FUNCTION "FC_GRP_81_R29" : VOID
TITLE =GROUP =81-R29
{ S7_language := '9(1) Angielski (Stany Zjednoczone)  11.01.2022  09:45:15' }
VERSION : 0.1


VAR_TEMP
  CL : "UDT_CABINET";	//CABINET LOCAL
  CR : "UDT_CABINET";	//CABINET REMOTE
  RelError : BOOL ;	//ERROR RELEASE
  RelErrorCL : BOOL ;	//ERROR RELEASE FROM CABINET LOCAL
  RelErrorCR : BOOL ;	//ERROR RELEASE FROM CABINET REMOTE
  RelControl : BOOL ;	//CONTROL RELEASE
  RelControlCL : BOOL ;	//CONTROL RELEASE FROM CABINET LOCAL
  RelControlCR : BOOL ;	//CONTROL RELEASE FROM CABINET REMOTE
  ErrorConfirm : BOOL ;	//ERROR CONFIRM
  AutoOn : BOOL ;	//AUTOMATIC ON
  AutoOff : BOOL ;	//AUTOMATIC OFF
  LAMP_ON : BOOL ;
  Setpoint_81FAN72_reached : BOOL ;
  Setpoint_81FAN72_div : BOOL ;
END_VAR
BEGIN
NETWORK
TITLE =GLOBAL SIGNALS
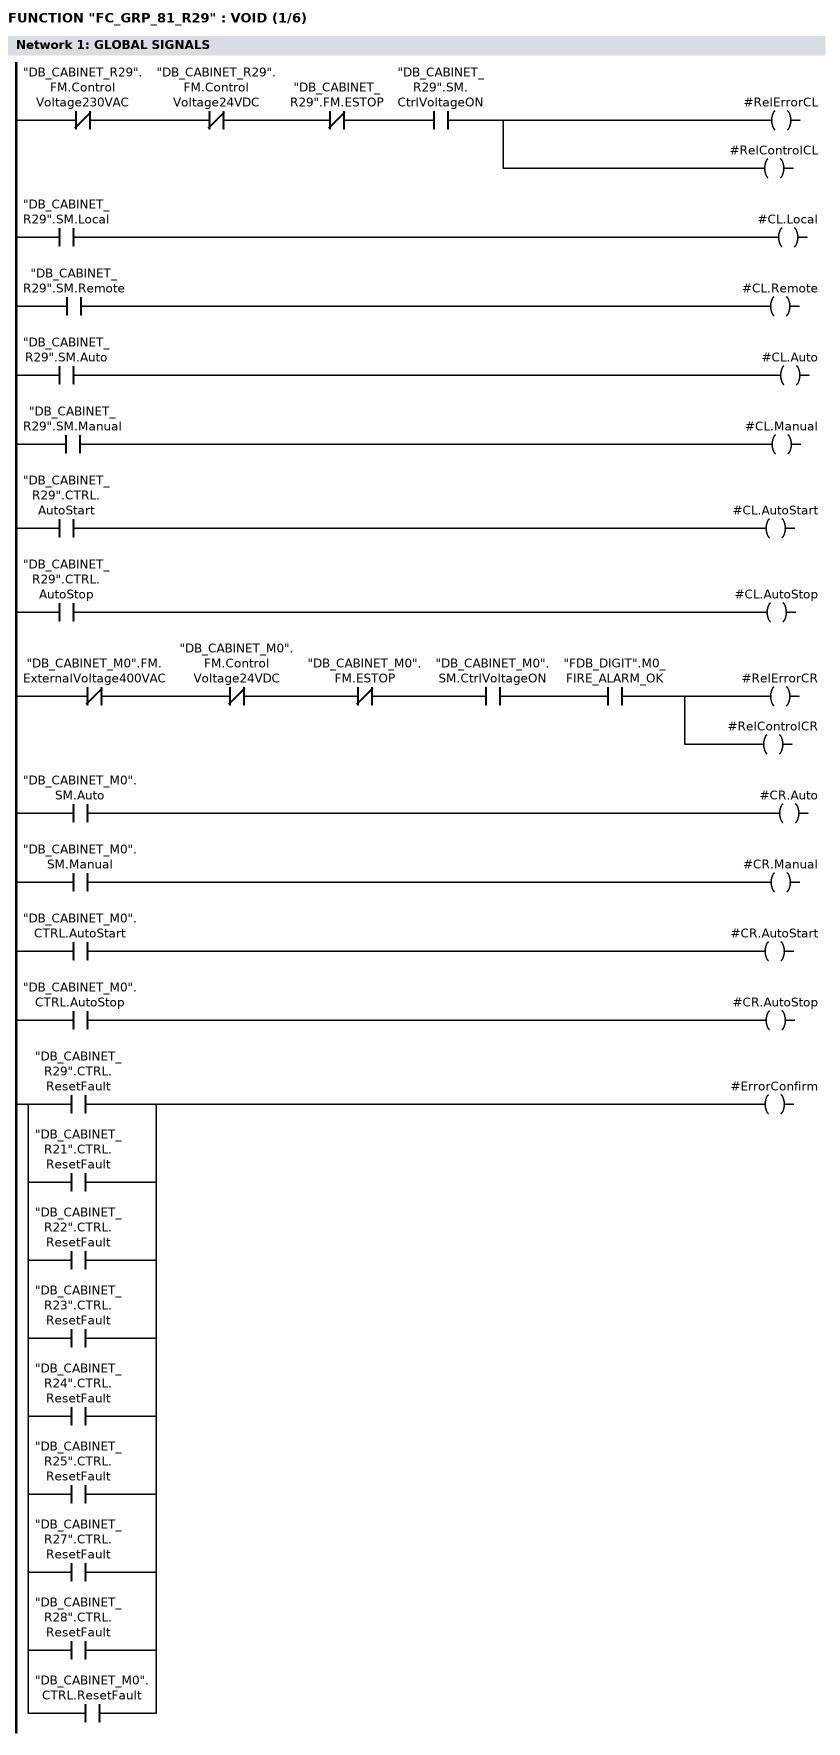
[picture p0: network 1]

// LOCAL
      UN    "DB_CABINET_R29".FM.ControlVoltage230VAC;
      UN    "DB_CABINET_R29".FM.ControlVoltage24VDC;
//      UN    "DB_CABINET_R29".FM.ControlVoltage230VAC_MS
      UN    "DB_CABINET_R29".FM.ESTOP;
      U     "DB_CABINET_R29".SM.CtrlVoltageON;
      =     #RelErrorCL;
      =     #RelControlCL;


      U     "DB_CABINET_R29".SM.Local;
      =     #CL.Local;
      U     "DB_CABINET_R29".SM.Remote;
      =     #CL.Remote;
      U     "DB_CABINET_R29".SM.Auto;
      =     #CL.Auto;
      U     "DB_CABINET_R29".SM.Manual;
      =     #CL.Manual;
      U     "DB_CABINET_R29".CTRL.AutoStart;
      =     #CL.AutoStart;
      U     "DB_CABINET_R29".CTRL.AutoStop;
      =     #CL.AutoStop;

// REMOTE
      UN    "DB_CABINET_M0".FM.ExternalVoltage400VAC;
      UN    "DB_CABINET_M0".FM.ControlVoltage24VDC;
//      UN    "DB_CABINET_M0".FM.ControlVoltage230VAC_MS
      UN    "DB_CABINET_M0".FM.ESTOP;
      U     "DB_CABINET_M0".SM.CtrlVoltageON;
      U     "FDB_DIGIT".M0_FIRE_ALARM_OK;
      =     #RelErrorCR;
      =     #RelControlCR;

      U     "DB_CABINET_M0".SM.Auto;
      =     #CR.Auto;
      U     "DB_CABINET_M0".SM.Manual;
      =     #CR.Manual;
      U     "DB_CABINET_M0".CTRL.AutoStart;
      =     #CR.AutoStart;
      U     "DB_CABINET_M0".CTRL.AutoStop;
      =     #CR.AutoStop;

      U     "DB_CABINET_R29".CTRL.ResetFault;
      O     "DB_CABINET_R21".CTRL.ResetFault;
      O     "DB_CABINET_R22".CTRL.ResetFault;
      O     "DB_CABINET_R23".CTRL.ResetFault;
      O     "DB_CABINET_R24".CTRL.ResetFault;
      O     "DB_CABINET_R25".CTRL.ResetFault;
      O     "DB_CABINET_R27".CTRL.ResetFault;
      O     "DB_CABINET_R28".CTRL.ResetFault;
      O     "DB_CABINET_M0".CTRL.ResetFault;
      =     #ErrorConfirm;

NETWORK
TITLE ==81FAN72-U1 CONTROL/ERROR RELEASE
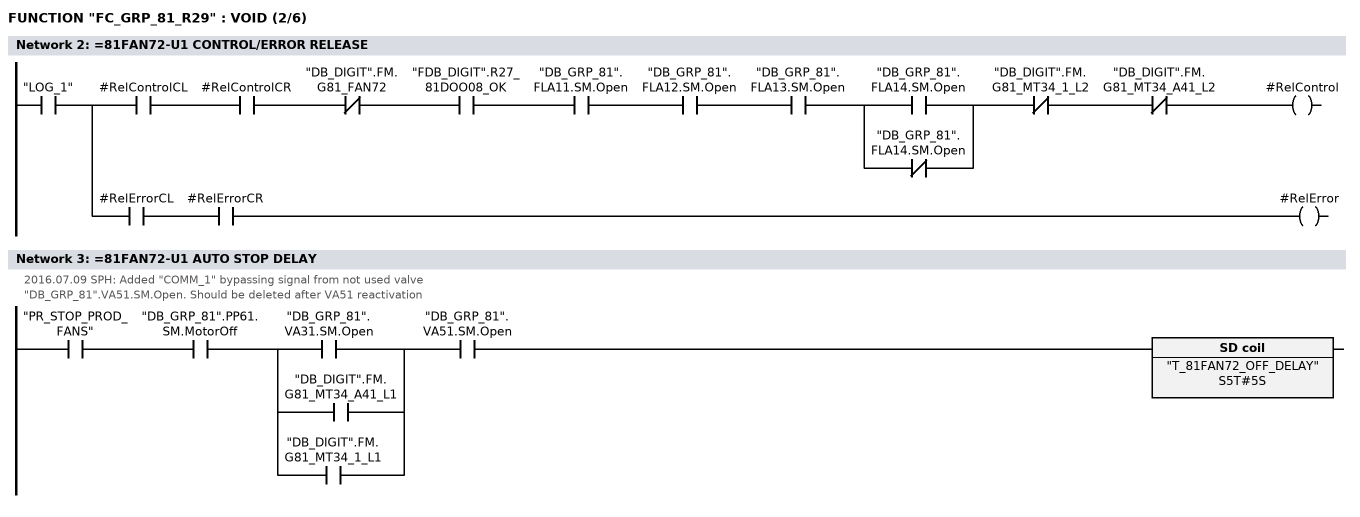
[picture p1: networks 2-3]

      U     "LOG_1";
      =     L      6.0;
      U     L      6.0;
      U     #RelControlCL;
      U     #RelControlCR;
      UN    "DB_DIGIT".FM.G81_FAN72;
      U     "FDB_DIGIT".R27_81DOO08_OK;
      U     "DB_GRP_81".FLA11.SM.Open;
      U     "DB_GRP_81".FLA12.SM.Open;
      U     "DB_GRP_81".FLA13.SM.Open;
      U(    ;
      O     "DB_GRP_81".FLA14.SM.Open;
      ON    "DB_GRP_81".FLA14.SM.Open;
      )     ;
      UN    "DB_DIGIT".FM.G81_MT34_1_L2;
      UN    "DB_DIGIT".FM.G81_MT34_A41_L2;
      =     #RelControl;
      U     L      6.0;
      U     #RelErrorCL;
      U     #RelErrorCR;
      =     #RelError;
NETWORK
TITLE ==81FAN72-U1 AUTO STOP DELAY
//2016.07.09 SPH: Added "COMM_1" bypassing signal from not used valve
//"DB_GRP_81".VA51.SM.Open. Should be deleted after VA51 reactivation
      U     "PR_STOP_PROD_FANS";
      U     "DB_GRP_81".PP61.SM.MotorOff;
      U(    ;
      O     "DB_GRP_81".VA31.SM.Open;
      O     "DB_DIGIT".FM.G81_MT34_A41_L1;
      O     "DB_DIGIT".FM.G81_MT34_1_L1;
      )     ;
      U     "DB_GRP_81".VA51.SM.Open;
      L     S5T#5S;
      SE    "T_81FAN72_OFF_DELAY";
      NOP   0;
      NOP   0;
      NOP   0;
      NOP   0;
NETWORK
TITLE ==81FAN72-U1 CONTROL SIGNALS
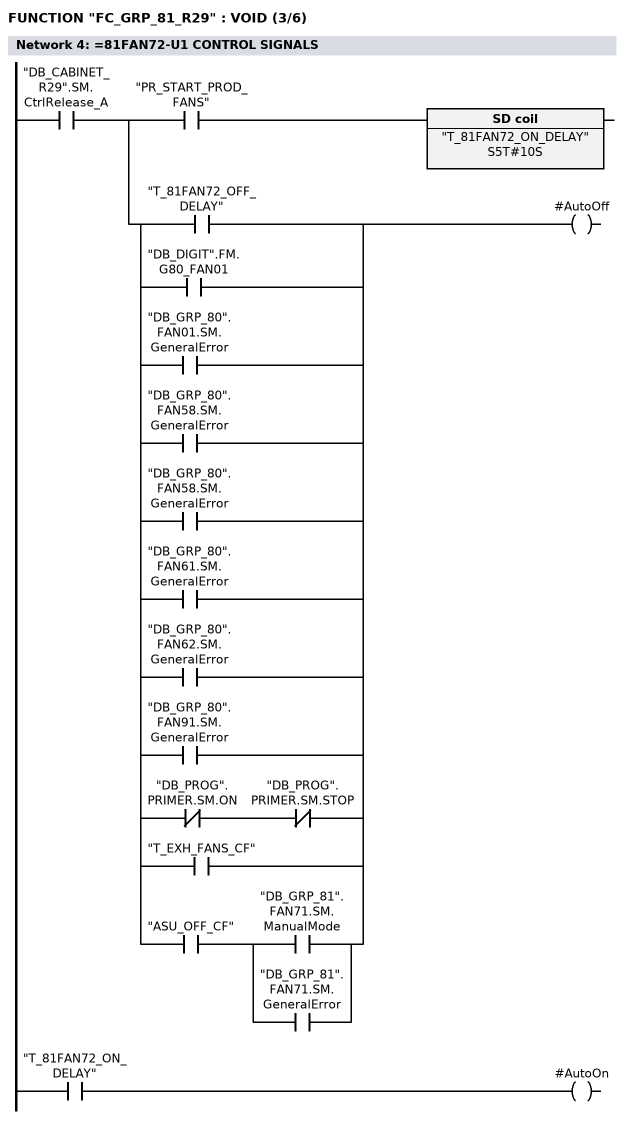
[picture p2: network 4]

      U     "DB_CABINET_R29".SM.CtrlRelease_A;
      =     L      6.0;
      U     L      6.0;
      U     "PR_START_PROD_FANS";
      L     S5T#10S;
      SE    "T_81FAN72_ON_DELAY";
      NOP   0;
      NOP   0;
      NOP   0;
      U     "T_81FAN72_ON_DELAY";
      =     #AutoOn;
      U     L      6.0;
      U(    ;
      O     "T_81FAN72_OFF_DELAY";
      O     "DB_DIGIT".FM.G80_FAN01;
      O     "DB_GRP_80".FAN01.SM.GeneralError;
      O     "DB_GRP_80".FAN58.SM.GeneralError;
      O     "DB_GRP_80".FAN58.SM.GeneralError;
      O     "DB_GRP_80".FAN61.SM.GeneralError;
      O     "DB_GRP_80".FAN62.SM.GeneralError;
      O     "DB_GRP_80".FAN91.SM.GeneralError;
      O     ;
      UN    "DB_PROG".PRIMER.SM.ON;
      UN    "DB_PROG".PRIMER.SM.STOP;
      O     "T_EXH_FANS_CF";
      O     ;
      U     "ASU_OFF_CF";
      U(    ;
      O     "DB_GRP_81".FAN71.SM.ManualMode;
      O     "DB_GRP_81".FAN71.SM.GeneralError;
      )     ;
      )     ;
      =     #AutoOff;
NETWORK
TITLE =SET POINT
//2.800000e+001
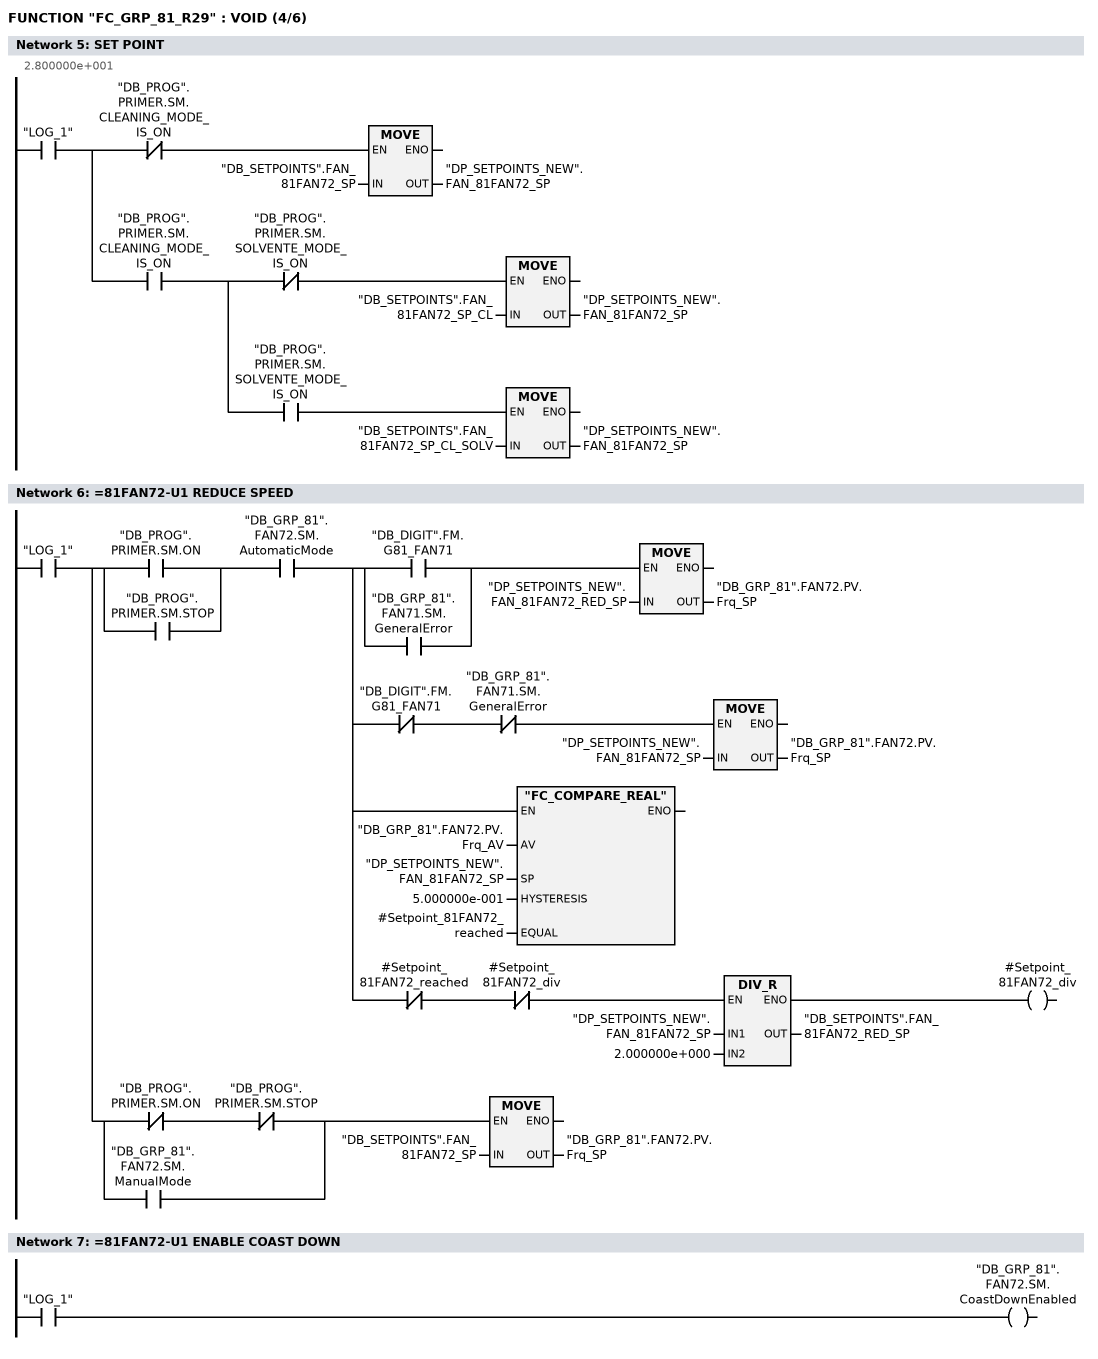
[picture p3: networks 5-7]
      U     "LOG_1";
      =     L      6.0;
      U     L      6.0;
      UN    "DB_PROG".PRIMER.SM.CLEANING_MODE_IS_ON;
      SPBNB _001;
      L     "DB_SETPOINTS".FAN_81FAN72_SP;
      T     "DP_SETPOINTS_NEW".FAN_81FAN72_SP;
_001: NOP   0;
      U     L      6.0;
      U     "DB_PROG".PRIMER.SM.CLEANING_MODE_IS_ON;
      =     L      6.1;
      U     L      6.1;
      UN    "DB_PROG".PRIMER.SM.SOLVENTE_MODE_IS_ON;
      SPBNB _002;
      L     "DB_SETPOINTS".FAN_81FAN72_SP_CL;
      T     "DP_SETPOINTS_NEW".FAN_81FAN72_SP;
_002: NOP   0;
      U     L      6.1;
      U     "DB_PROG".PRIMER.SM.SOLVENTE_MODE_IS_ON;
      SPBNB _003;
      L     "DB_SETPOINTS".FAN_81FAN72_SP_CL_SOLV;
      T     "DP_SETPOINTS_NEW".FAN_81FAN72_SP;
_003: NOP   0;
NETWORK
TITLE ==81FAN72-U1 REDUCE SPEED

      U     "LOG_1";
      =     L      6.0;
      U     L      6.0;
      U(    ;
      O     "DB_PROG".PRIMER.SM.ON;
      O     "DB_PROG".PRIMER.SM.STOP;
      )     ;
      U     "DB_GRP_81".FAN72.SM.AutomaticMode;
      =     L      6.1;
      U     L      6.1;
      U(    ;
      O     "DB_DIGIT".FM.G81_FAN71;
      O     "DB_GRP_81".FAN71.SM.GeneralError;
      )     ;
      SPBNB _004;
      L     "DP_SETPOINTS_NEW".FAN_81FAN72_RED_SP;
      T     "DB_GRP_81".FAN72.PV.Frq_SP;
_004: NOP   0;
      U     L      6.1;
      UN    "DB_DIGIT".FM.G81_FAN71;
      UN    "DB_GRP_81".FAN71.SM.GeneralError;
      SPBNB _005;
      L     "DP_SETPOINTS_NEW".FAN_81FAN72_SP;
      T     "DB_GRP_81".FAN72.PV.Frq_SP;
_005: NOP   0;
      U     L      6.1;
      SPBNB _006;
      CALL "FC_COMPARE_REAL" (
           AV                       := "DB_GRP_81".FAN72.PV.Frq_AV,
           SP                       := "DP_SETPOINTS_NEW".FAN_81FAN72_SP,
           HYSTERESIS               := 5.000000e-001,
           EQUAL                    := #Setpoint_81FAN72_reached);
_006: NOP   0;
      U     L      6.1;
      UN    #Setpoint_81FAN72_reached;
      UN    #Setpoint_81FAN72_div;
      SPBNB _007;
      L     "DP_SETPOINTS_NEW".FAN_81FAN72_SP;
      L     2.000000e+000;
      /R    ;
      T     "DB_SETPOINTS".FAN_81FAN72_RED_SP;
      UN    OV;
      SAVE  ;
      CLR   ;
_007: U     BIE;
      =     #Setpoint_81FAN72_div;
      U     L      6.0;
      U(    ;
      UN    "DB_PROG".PRIMER.SM.ON;
      UN    "DB_PROG".PRIMER.SM.STOP;
      O     "DB_GRP_81".FAN72.SM.ManualMode;
      )     ;
      SPBNB _008;
      L     "DB_SETPOINTS".FAN_81FAN72_SP;
      T     "DB_GRP_81".FAN72.PV.Frq_SP;
_008: NOP   0;
NETWORK
TITLE ==81FAN72-U1 ENABLE COAST DOWN

      U     "LOG_1";
      =     "DB_GRP_81".FAN72.SM.CoastDownEnabled;
NETWORK
TITLE =RESET USING ESTOP ON THE CABINET
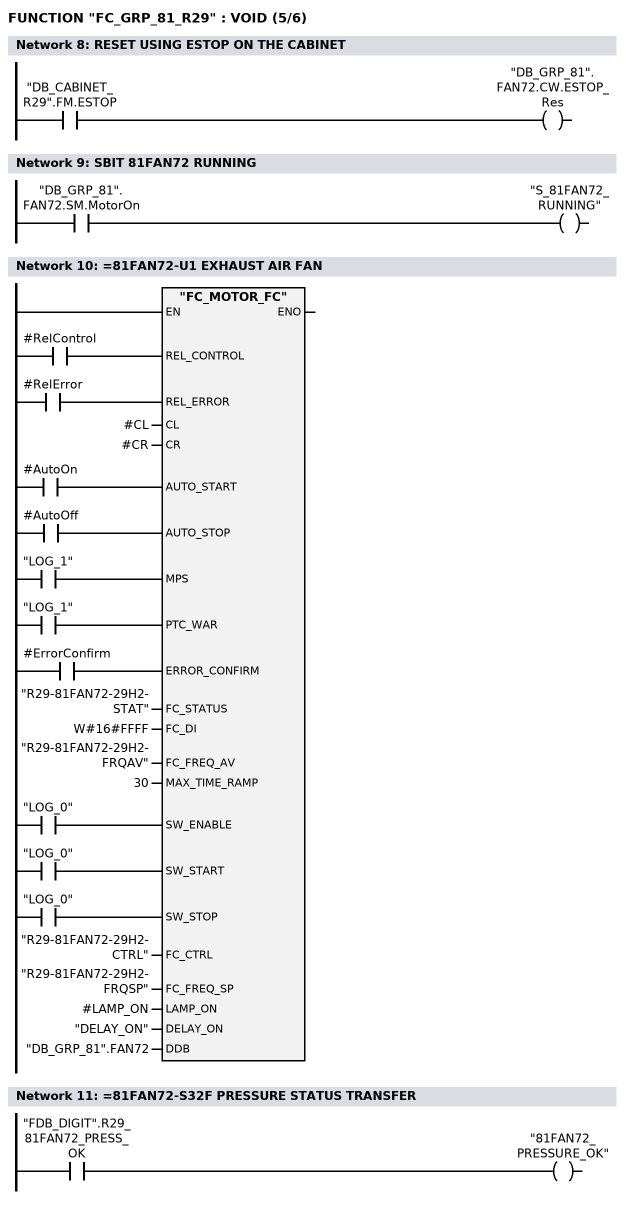
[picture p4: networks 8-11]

      U     "DB_CABINET_R29".FM.ESTOP;
      =     "DB_GRP_81".FAN72.CW.ESTOP_Res;
NETWORK
TITLE =SBIT 81FAN72 RUNNING

      U     "DB_GRP_81".FAN72.SM.MotorOn;
      =     "S_81FAN72_RUNNING";
NETWORK
TITLE ==81FAN72-U1 EXHAUST AIR FAN

      U     #RelControl;
      =     L      6.0;
      BLD   103;
      U     #RelError;
      =     L      6.1;
      BLD   103;
      U     #AutoOn;
      =     L      6.2;
      BLD   103;
      U     #AutoOff;
      =     L      6.3;
      BLD   103;
      U     "LOG_1";
      =     L      6.4;
      BLD   103;
      U     "LOG_1";
      =     L      6.5;
      BLD   103;
      U     #ErrorConfirm;
      =     L      6.6;
      BLD   103;
      U     "LOG_0";
      =     L      6.7;
      BLD   103;
      U     "LOG_0";
      =     L      7.0;
      BLD   103;
      U     "LOG_0";
      =     L      7.1;
      BLD   103;
      CALL "FC_MOTOR_FC" (
           REL_CONTROL              := L      6.0,
           REL_ERROR                := L      6.1,
           CL                       := #CL,
           CR                       := #CR,
           AUTO_START               := L      6.2,
           AUTO_STOP                := L      6.3,
           MPS                      := L      6.4,
           PTC_WAR                  := L      6.5,
           ERROR_CONFIRM            := L      6.6,
           FC_STATUS                := "R29-81FAN72-29H2-STAT",
           FC_DI                    := W#16#FFFF,
           FC_FREQ_AV               := "R29-81FAN72-29H2-FRQAV",
           MAX_TIME_RAMP            := 30,
           SW_ENABLE                := L      6.7,
           SW_START                 := L      7.0,
           SW_STOP                  := L      7.1,
           FC_CTRL                  := "R29-81FAN72-29H2-CTRL",
           FC_FREQ_SP               := "R29-81FAN72-29H2-FRQSP",
           LAMP_ON                  := #LAMP_ON,
           DELAY_ON                 := "DELAY_ON",
           DDB                      := "DB_GRP_81".FAN72);
      NOP   0;
NETWORK
TITLE ==81FAN72-S32F PRESSURE STATUS TRANSFER

      U     "FDB_DIGIT".R29_81FAN72_PRESS_OK;
      =     "81FAN72_PRESSURE_OK";
NETWORK
TITLE ==81FAN72-S32F PRESSURE MONITORING
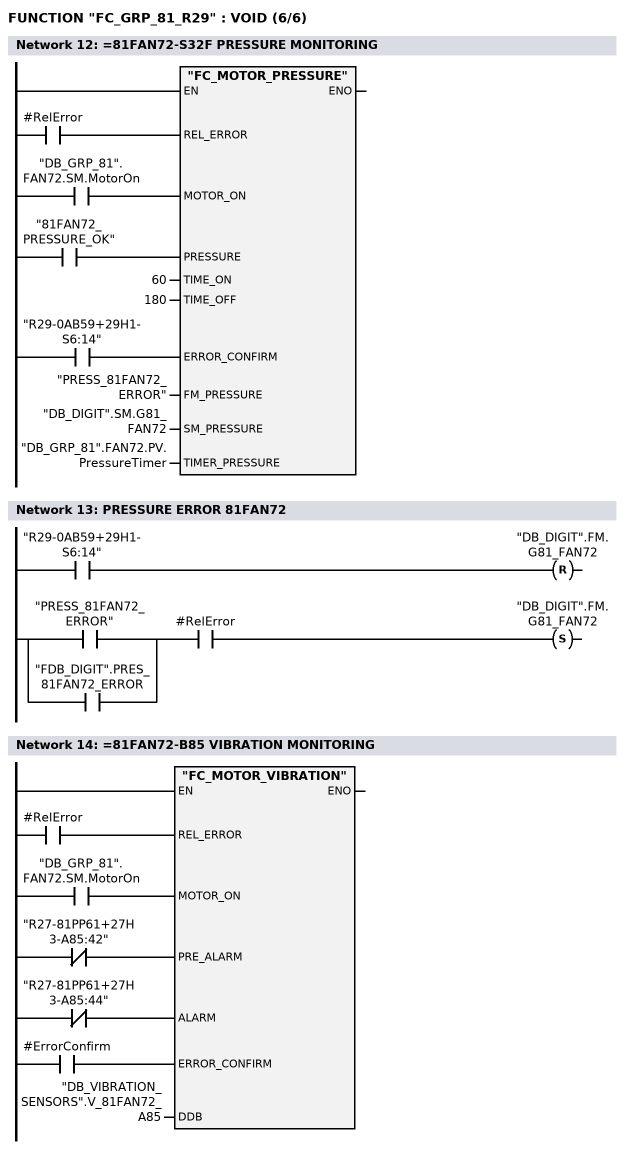
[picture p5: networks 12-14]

      U     #RelError;
      =     L      6.0;
      BLD   103;
      U     "DB_GRP_81".FAN72.SM.MotorOn;
      =     L      6.1;
      BLD   103;
      U     "81FAN72_PRESSURE_OK";
      =     L      6.2;
      BLD   103;
      U     "R29-0AB59+29H1-S6:14";
      =     L      6.3;
      BLD   103;
      CALL "FC_MOTOR_PRESSURE" (
           REL_ERROR                := L      6.0,
           MOTOR_ON                 := L      6.1,
           PRESSURE                 := L      6.2,
           TIME_ON                  := 60,
           TIME_OFF                 := 180,
           ERROR_CONFIRM            := L      6.3,
           FM_PRESSURE              := "PRESS_81FAN72_ERROR",
           SM_PRESSURE              := "DB_DIGIT".SM.G81_FAN72,
           TIMER_PRESSURE           := "DB_GRP_81".FAN72.PV.PressureTimer);
      NOP   0;
NETWORK
TITLE =PRESSURE ERROR 81FAN72

      U     "R29-0AB59+29H1-S6:14";
      R     "DB_DIGIT".FM.G81_FAN72;
      U(    ;
      O     "PRESS_81FAN72_ERROR";
      O     "FDB_DIGIT".PRES_81FAN72_ERROR;
      )     ;
      U     #RelError;
      S     "DB_DIGIT".FM.G81_FAN72;
      NOP   0;
NETWORK
TITLE ==81FAN72-B85 VIBRATION MONITORING

      U     #RelError;
      =     L      6.0;
      BLD   103;
      U     "DB_GRP_81".FAN72.SM.MotorOn;
      =     L      6.1;
      BLD   103;
      UN    "R27-81PP61+27H3-A85:42";
      =     L      6.2;
      BLD   103;
      UN    "R27-81PP61+27H3-A85:44";
      =     L      6.3;
      BLD   103;
      U     #ErrorConfirm;
      =     L      6.4;
      BLD   103;
      CALL "FC_MOTOR_VIBRATION" (
           REL_ERROR                := L      6.0,
           MOTOR_ON                 := L      6.1,
           PRE_ALARM                := L      6.2,
           ALARM                    := L      6.3,
           ERROR_CONFIRM            := L      6.4,
           DDB                      := "DB_VIBRATION_SENSORS".V_81FAN72_A85);
      NOP   0;
NETWORK
TITLE =END



END_FUNCTION

